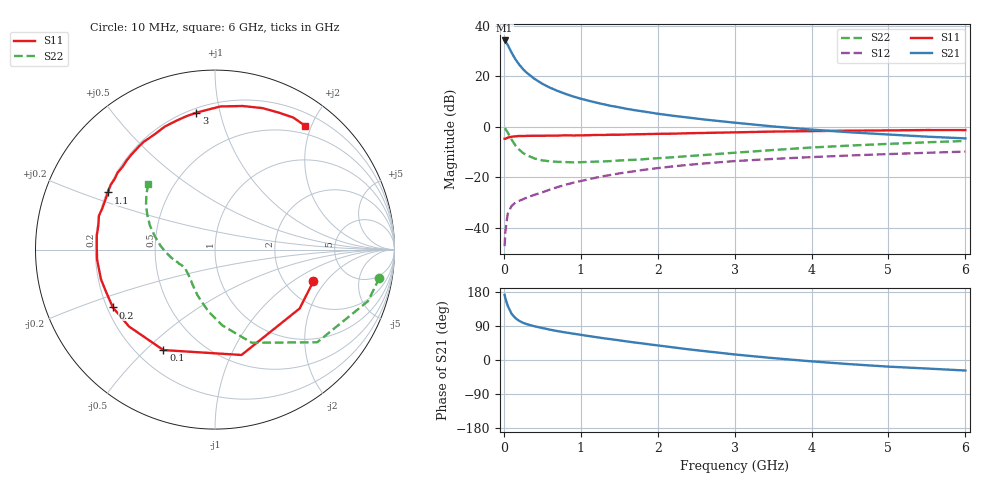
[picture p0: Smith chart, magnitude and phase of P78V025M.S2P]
! SIEMENS Small Signal Semiconductors
! BFP196
! Si NPN RF Bipolar Junction Transistor in SOT143
! VCE = 8 V  IC = 25 mA
! Common Emitter S-Parameters:  May  1996
# GHz  S  MA  R  50
!  f  S11  S21  S12  S22
! GHz  MAG  ANG  MAG  ANG  MAG  ANG  MAG  ANG
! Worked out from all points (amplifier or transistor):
!   36 points, 10 MHz to 6 GHz, reference 50 ohm
!   highest |S21| = 34.1 dB at 10 MHz (marker M1)
!   |S21| within 3 dB of that: start of sweep to 70.58 MHz
!   unconditionally stable (mu >= 1): 659.2 MHz to 4.093 GHz
!   at 250 MHz: K = 0.63, MSG = 25.7 dB, |S12| = -28.8 dB
!   at 1.4 GHz: K = 1.09, MAG = 11.8 dB, |S12| = -19.1 dB
!   at 6 GHz: K = 0.97, MSG = 2.6 dB, |S12| = -9.9 dB
!   S11 on the Smith chart (normalised r, x): 10 MHz: 2.84, -1.50; 100 MHz: 0.31, -0.57; 200 MHz: 0.22, -0.25; 1.1 GHz: 0.20, +0.24; 3 GHz: 0.23, +0.85; 6 GHz: 0.38, +1.91
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0.01  0.576 -17.9  50.79 171.8  0.0043 81.7  0.9297 -9.7
0.02  0.5744 -34.9  48.65 162.9  0.0084 77.2  0.8998 -18.6
0.05  0.6054 -75.9  41.46 143.1  0.0187 59.9  0.7686 -42.2
0.1  0.6293 -117.2  29.33 122.2  0.0269 48.0  0.5579 -68.5
0.15  0.6428 -138.2  21.56 110.5  0.0313 42.4  0.4247 -84.4
0.2  0.6539 -150.5  16.92 103.3  0.034 42.1  0.3494 -95.6
0.25  0.6511 -159.3  13.7 98.1  0.0365 42.7  0.2999 -104.4
0.3  0.6565 -165.4  11.58 94.5  0.0394 44.9  0.2714 -111.2
0.4  0.6591 -175.1  8.809 88.9  0.0448 47.3  0.2339 -121.9
0.5  0.6589 179.1  7.057 84.4  0.05 50.3  0.2148 -129.4
0.6  0.6633 173.2  5.9 80.1  0.0569 51.5  0.2054 -135.2
0.8  0.6737 163.8  4.449 72.8  0.0704 53.8  0.1986 -143.4
0.9  0.6685 160.0  3.955 69.6  0.0775 54.0  0.1964 -146.5
1.1  0.6765 151.9  3.258 63.3  0.0907 53.8  0.2003 -150.8
1.3  0.6839 144.7  2.763 57.3  0.1049 52.7  0.2049 -154.9
1.6  0.6982 135.1  2.247 49.0  0.1249 50.4  0.2177 -159.9
2.2  0.7249 117.7  1.64 33.4  0.1633 43.8  0.2477 -169.5
3  0.77 97.7  1.197 14.6  0.2077 33.5  0.3042 176.0
3.5  0.798 87.9  1.008 5.0  0.2295 27.1  0.344 167.4
4.5  0.8316 71.4  0.772 -11.0  0.2687 15.9  0.4217 153.2
5.5  0.8552 59.3  0.633 -22.5  0.3036 5.4  0.4894 141.4
6  0.8536 53.8  0.585 -27.8  0.3202 -0.2  0.5204 135.7
